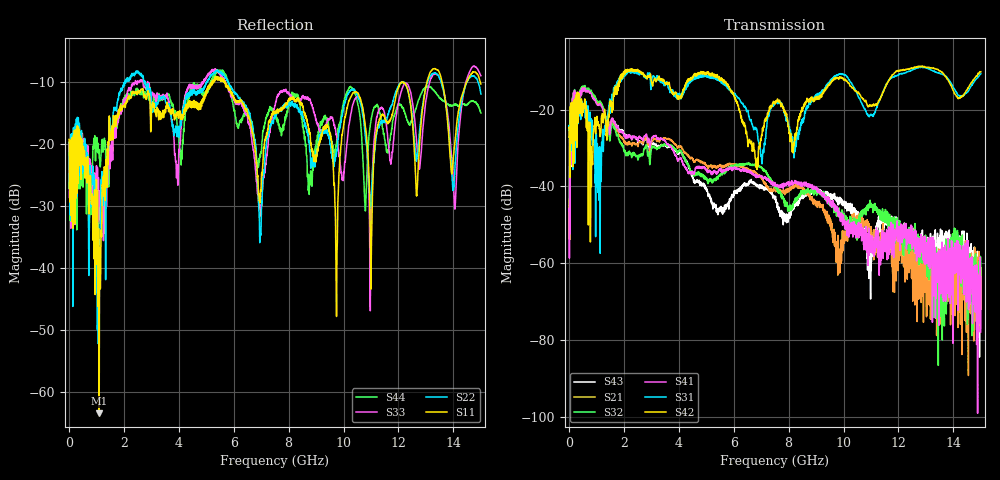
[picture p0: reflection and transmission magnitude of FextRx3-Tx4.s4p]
! FILE: N:\QM 2007\Prüfprotokolle\Highspeed\Konfektionierte Ltg\L45593-D106\D30\8216\0002\Fext\FextRx3-Tx4.s4p
# MHz S DB R 50.00
! FREQ  S11  S12  S13  S14
!  S21  S22  S23  S24
!  S31  S32  S33  S34
!  S41  S42  S43  S44
!  DB  ANG  DB  ANG  DB  ANG  DB  ANG
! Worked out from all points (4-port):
!   2999 points, 10 MHz to 15 GHz, reference 50 ohm
!   strongest paths, dB at 10 MHz, 3.755 GHz, 7.505 GHz, 11.26 GHz, 15 GHz:
!     S42: -24.8, -15.4, -18.6, -18.2, -10.2
!     S31: -25.3, -15.7, -18.2, -18.4, -10.7
!     S41: -45.7, -30.0, -39.8, -51.5, -63.5
!     S32: -47.4, -29.4, -39.5, -46.8, -71.2
!     S21: -43.6, -28.2, -40.3, -55.0, -61.2
!     S43: -47.0, -29.7, -43.3, -49.0, -66.6
!   lowest |S11| = -63.4 dB at 1.105 GHz (marker M1), VSWR 1.00, Z = 49.9 + j0.038 ohm
!   |S11| at or under -10 dB: start of sweep to 5.213 GHz; 5.69 GHz to 13.04 GHz (7.345 GHz wide, 78.5 % of centre); 13.59 GHz to 14.48 GHz (893.8 MHz wide, 6.37 % of centre)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
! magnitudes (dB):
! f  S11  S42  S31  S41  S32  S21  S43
! 10 MHz  -19.3  -24.8  -25.3  -45.7  -47.4  -43.6  -47.0
! 190 MHz  -20.3  -19.8  -19.8  -21.8  -21.8  -22.1  -22.0
! 1.105 GHz  -63.4  -25.0  -36.7  -18.8  -18.0  -18.5  -18.4
! 2.475 GHz  -11.8  -9.9  -10.4  -27.4  -31.9  -29.0  -27.6
! 6.83 GHz  -23.0  -33.9  -24.9  -37.7  -34.5  -36.6  -39.6
! 9.745 GHz  -47.8  -11.8  -11.1  -46.0  -47.7  -56.2  -43.2
! 15 GHz  -10.3  -10.2  -10.7  -63.5  -71.2  -61.2  -66.6
